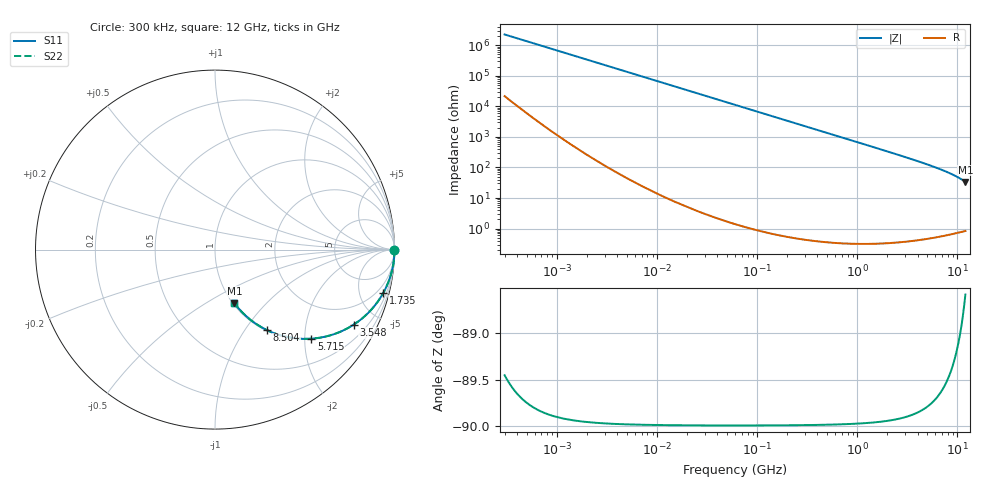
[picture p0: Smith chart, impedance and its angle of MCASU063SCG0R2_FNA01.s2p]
! MCASU063SCG0R2_FNA01  S-PARAMETER MODEL  ( Standard Model )
! Model Generated by TAIYO YUDEN Corporation (http://www.ty-top.com)
! Version 1.0
! TAIYO YUDEN Control No. 230609
! Copyright(c) 2023 TAIYO YUDEN CO.,LTD. All Rights Reserved.
! Product Description (link to TY-COMPAS)
! https://ds.yuden.co.jp/TYCOMPAS/or/detail?pn=MCASU063SCG0R2BFNA01&u=M
! Products Name : Multilayer Ceramic Capacitors
! Characteristics :
!  Capacitance : 0.2 [pF] , Rated Voltage : 50 [V] , TCC : CG / C0G
!  Case Size : 0.6 x 0.3 / 0.024 x 0.012 [mm/inch] , Thickness : 0.3 / 0.012 [mm/inch]
!  (Conditions: Temperature = 25 [degC] , DC Bias Voltage = 0 [V])
! External Node Assignments :
!  1  o---| |---o  2
! GND o---------o GND
! Frequency Range : 0.3MHz  -  12000MHz  [ 401 STEP ]
# MHZ S RI R 50
! Freq[MHz].  S11 Real  S11 Imag  S21 Real  S21 Imag  S12 Real  S12 Imag  S22 Real  S22 Imag
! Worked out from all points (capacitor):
!   401 points, 300 kHz to 12 GHz, reference 50 ohm
!   read as one part in series: C = 235 fF near 316.3 kHz
!   lowest |Z| = 33.8 ohm at 12 GHz (marker M1)
!   S11 on the Smith chart (normalised r, x): 300 kHz: open; 1.735 GHz: 1.01, -7.74; 3.548 GHz: 1.01, -3.68; 5.715 GHz: 1.01, -2.15; 8.504 GHz: 1.01, -1.27; 12 GHz: 1.02, -0.68
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0.3  1 -4.43e-05  4.26e-07 4.43e-05  4.26e-07 4.43e-05  1 -4.43e-05
0.629891  1 -9.3e-05  3.02e-07 9.3e-05  3.02e-07 9.3e-05  1 -9.3e-05
0.681995  1 -0.000101  2.94e-07 0.000101  2.94e-07 0.000101  1 -0.000101
1.769972  1 -0.000261  2.96e-07 0.000261  2.96e-07 0.000261  1 -0.000261
10.44266  1 -0.00154  2.69e-06 0.00154  2.69e-06 0.00154  1 -0.00154
60  0.9999 -0.00886  7.96e-05 0.00886  7.96e-05 0.00886  0.9999 -0.00886
164.1901  0.9994 -0.0242  0.000591 0.0242  0.000591 0.0242  0.9994 -0.0242
353.9943  0.9973 -0.0522  0.00274 0.0522  0.00274 0.0522  0.9973 -0.0522
570.2811  0.9929 -0.0837  0.00708 0.0837  0.00708 0.0837  0.9929 -0.0837
848.5281  0.9844 -0.1236  0.0156 0.1236  0.0156 0.1236  0.9844 -0.1236
1229.528  0.9677 -0.1764  0.0323 0.1764  0.0323 0.1764  0.9677 -0.1764
1735.023  0.9372 -0.2421  0.0628 0.2421  0.0628 0.2421  0.9372 -0.2421
2088.533  0.9109 -0.2843  0.0891 0.2843  0.0891 0.2843  0.9109 -0.2843
2722.03  0.8555 -0.3509  0.1445 0.3509  0.1445 0.3509  0.8555 -0.3509
3547.679  0.7718 -0.4186  0.2282 0.4186  0.2282 0.4186  0.7718 -0.4186
4502.883  0.6677 -0.4695  0.3323 0.4695  0.3323 0.4695  0.6677 -0.4695
5715.274  0.5369 -0.4963  0.4631 0.4963  0.4631 0.4963  0.5369 -0.4963
7064.448  0.4059 -0.4877  0.5941 0.4877  0.5941 0.4877  0.4059 -0.4877
8503.825  0.29 -0.4487  0.71 0.4487  0.71 0.4487  0.29 -0.4487
9454.42  0.2275 -0.4128  0.7725 0.4128  0.7725 0.4128  0.2275 -0.4128
10511.28  0.1702 -0.3675  0.8298 0.3675  0.8298 0.3675  0.1702 -0.3675
12000  0.1086 -0.299  0.8914 0.299  0.8914 0.299  0.1086 -0.299
